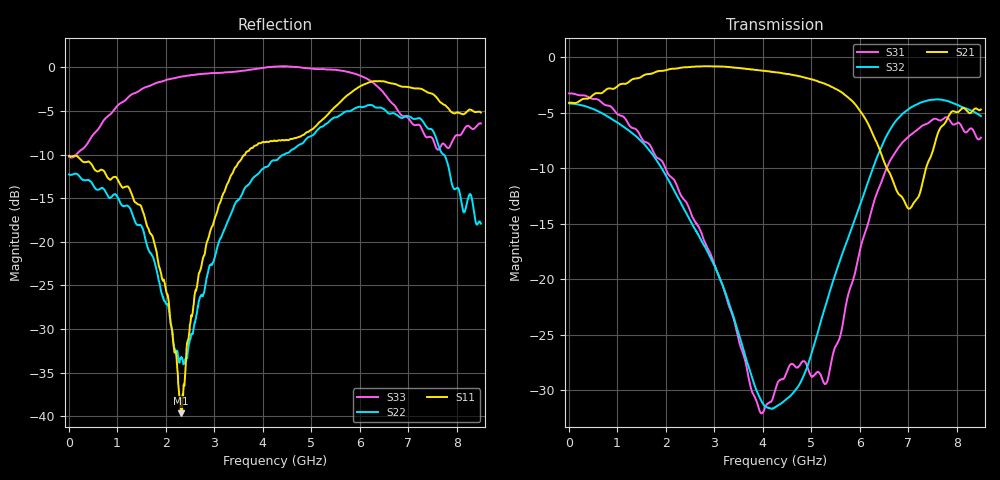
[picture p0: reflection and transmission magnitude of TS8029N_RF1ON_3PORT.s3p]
!Created with skrf (http://scikit-rf.org).
# GHz S RI R 50.0
!freq ReS11 ImS11 ReS12 ImS12 ReS13 ImS13
! ReS21 ImS21 ReS22 ImS22 ReS23 ImS23
! ReS31 ImS31 ReS32 ImS32 ReS33 ImS33
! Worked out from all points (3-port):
!   1601 points, 10 MHz to 8.5 GHz, reference 50 ohm
!   strongest paths, dB at 10 MHz, 2.132 GHz, 4.255 GHz, 6.378 GHz, 8.5 GHz:
!     S21: -4.1, -1.1, -1.4, -7.9, -4.7
!     S32: -4.2, -11.7, -31.6, -8.8, -5.3
!     S31: -3.3, -10.9, -30.1, -12.0, -7.3
!   lowest |S11| = -39.6 dB at 2.318 GHz (marker M1), VSWR 1.02, Z = 49 + j0.156 ohm
!   |S11| at or under -10 dB: start of sweep to 3.635 GHz
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0.01  -0.3107 0.0039  0.6231 0.000121  0.6861 -0.00705
      0.623 8.65e-05  -0.2435 0.00298  0.619 -0.00747
      0.686 -0.00719  0.6189 -0.00759  -0.3066 0.0112
0.9916563  -0.1598 0.1691  0.7267 -0.1003  0.3116 -0.4617
           0.727 -0.1007  -0.0829 0.1638  0.2503 -0.443
           0.3112 -0.4618  0.2508 -0.4429  0.3636 0.4727
1.761062  -0.0368 0.0928  0.7716 -0.3569  -0.0259 -0.3672
          0.7714 -0.357  0.0473 0.063  -0.1056 -0.3399
          -0.0258 -0.3675  -0.1059 -0.3401  0.8023 -0.0402
2.318219  -0.0103 0.00159  0.6912 -0.5699  -0.1117 -0.2098
          0.6911 -0.5702  0.0119 -0.0182  -0.1604 -0.1492
          -0.1115 -0.21  -0.1607 -0.1492  0.7331 -0.4937
3.124769  -0.119 -0.1184  0.4357 -0.7945  -0.0805 -0.059
          0.4355 -0.7947  -0.1002 -0.0281  -0.0999 -0.00399
          -0.0804 -0.0589  -0.0997 -0.00407  0.1749 -0.9135
4.255  -0.3414 -0.1663  -0.0387 -0.8537  0.00457 -0.031
       -0.0394 -0.8531  -0.2899 0.0387  0.0113 0.0239
       0.00443 -0.031  0.0113 0.0239  -0.6032 -0.8075
5.257881  -0.5077 0.0194  -0.3915 -0.653  -0.0334 -0.0072
          -0.3909 -0.6531  -0.2173 0.4077  0.0431 0.0566
          -0.0334 -0.00721  0.0432 0.0565  -0.9751 0.0557
6.409338  -0.5473 0.6294  -0.3457 -0.1692  0.158 0.2071
          -0.3454 -0.1695  0.1653 0.5634  0.3676 0.0785
          0.1581 0.207  0.3676 0.0782  -0.4101 0.6373
7.513038  0.1006 0.6945  -0.059 -0.3756  0.3741 -0.3673
          -0.059 -0.3761  0.4303 -0.0349  0.1215 -0.6317
          0.375 -0.3668  0.1222 -0.6306  0.244 0.3
8.5  0.1776 0.521  -0.3564 -0.4578  -0.1457 -0.4081
     -0.3573 -0.4571  0.127 -0.00579  -0.4361 -0.3216
     -0.1463 -0.4081  -0.4357 -0.3229  0.4438 0.174
